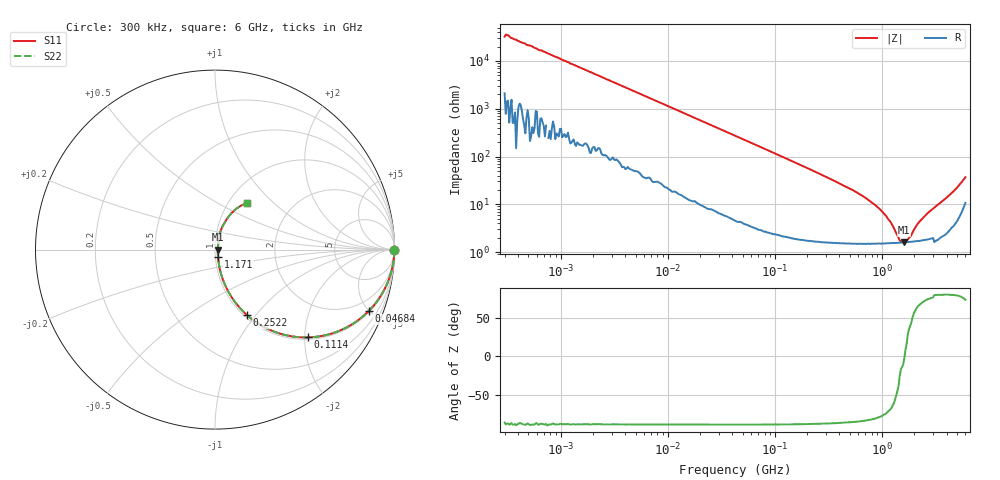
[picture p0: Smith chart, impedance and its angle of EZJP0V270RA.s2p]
!*** S-Parameter ***
!Copyright  (C)  Panasonic Corporation
!Multilaryer Varistors, Chip Type  Port assignments : Series-thru
!  1  o---GGG---o  2
!Parts No. : EZJP0V270RA  GND o---------o GND
# HZ S RI R 50
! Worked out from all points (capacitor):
!   401 points, 300 kHz to 6 GHz, reference 50 ohm
!   read as one part in series: C = 15 pF near 315.2 kHz
!   lowest |Z| = 1.59 ohm at 1.615 GHz (marker M1)
!   series resonance near 1.625 GHz, so ESL is about 640 pH
!   S11 on the Smith chart (normalised r, x): 300 kHz: open; 46.84 MHz: 1.09, -4.95; 111.4 MHz: 1.04, -2.08; 252.2 MHz: 1.03, -0.90; 1.171 GHz: 1.03, -0.09; 6 GHz: 1.21, +0.70
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300000  0.9998 -0.00309  0.000211 0.00309  0.000211 0.00309  0.9998 -0.00309
323131.3  0.9999 -0.00286  0.00013 0.00286  0.00013 0.00286  0.9999 -0.00286
1575955  0.9994 -0.0142  0.000551 0.0142  0.000551 0.0142  0.9994 -0.0142
8278779  0.9932 -0.0722  0.00675 0.0722  0.00675 0.0722  0.9932 -0.0722
2.284662e7  0.9592 -0.1898  0.0408 0.1898  0.0408 0.1898  0.9592 -0.1898
4.348994e7  0.8725 -0.3254  0.1275 0.3254  0.1275 0.3254  0.8725 -0.3254
4.68432e7  0.8554 -0.3431  0.1446 0.3431  0.1446 0.3431  0.8554 -0.3431
6.961258e7  0.7314 -0.4345  0.2686 0.4345  0.2686 0.4345  0.7314 -0.4345
1.11426e8  0.5196 -0.4891  0.4804 0.4891  0.4804 0.4891  0.5196 -0.4891
2.228737e8  0.2158 -0.3954  0.7842 0.3954  0.7842 0.3954  0.2158 -0.3954
2.522445e8  0.1778 -0.3645  0.8222 0.3645  0.8222 0.3645  0.1778 -0.3645
3.938837e8  0.0837 -0.2506  0.9163 0.2506  0.9163 0.2506  0.0837 -0.2506
6.790858e8  0.0336 -0.1352  0.9664 0.1352  0.9664 0.1352  0.0336 -0.1352
9.140197e8  0.0217 -0.0818  0.9783 0.0818  0.9783 0.0818  0.0217 -0.0818
1.170796e9  0.0168 -0.0418  0.9832 0.0418  0.9832 0.0418  0.0168 -0.0418
1.463034e9  0.0155 -0.00723  0.9845 0.00723  0.9845 0.00723  0.0155 -0.00723
1.615343e9  0.0157 -0.000694  0.9843 0.000694  0.9843 0.000694  0.0157 -0.000694
1.783508e9  0.0161 0.0109  0.9839 -0.0109  0.9839 -0.0109  0.0161 0.0109
2.174181e9  0.018 0.0351  0.982 -0.0351  0.982 -0.0351  0.018 0.0351
2.522384e9  0.0204 0.0524  0.9796 -0.0524  0.9796 -0.0524  0.0204 0.0524
4.457798e9  0.056 0.1529  0.944 -0.1529  0.944 -0.1529  0.056 0.1529
6e9  0.1793 0.2606  0.8207 -0.2606  0.8207 -0.2606  0.1793 0.2606
